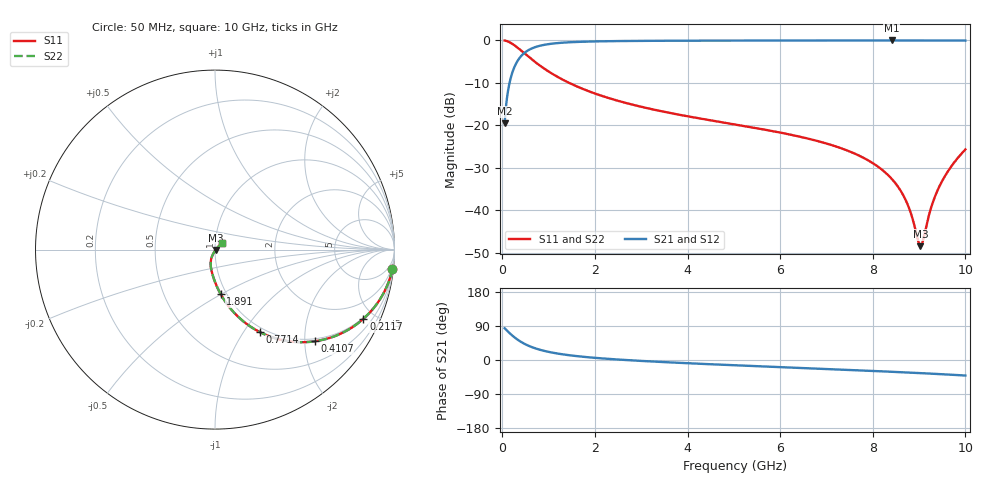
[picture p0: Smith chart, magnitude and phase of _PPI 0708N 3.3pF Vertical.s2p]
! S-Parameter data specifications (vertical orientation):
! Substrate: 40-mil Rogers 3003C, Substrate thickness, H=1.016mm, Dielectric constant, Er=3, Conductor thickness, T_mtl=0.043mm, Loss Tangent, Tand=0.003
! PCB Mounting Pad Footprint: Pad width, PadW=2.54mm , Pad length, PadL=0.51mm , Pad gap, PadG (edge-to-edge)=0.71mm , Reference planes=1.73mm apart
! Created Tue Jan 16 08:45:03 2018
# GHz S MA R 50
! 2 Port Network Data from SP1.SP block
! freq  magS11  angS11  magS21  angS21  magS12  angS12  magS22  angS22
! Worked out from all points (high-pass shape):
!   801 points, 50 MHz to 10 GHz, reference 50 ohm
!   highest |S21| = -0.03 dB at 8.408 GHz (marker M1); lowest = -19.5 dB at 50 MHz (marker M2)
!   |S21| within 3 dB of the highest: 470.5 MHz to end of sweep
!   lowest |S11| = -48.5 dB at 9.03 GHz (marker M3), VSWR 1.01, Z = 50.3 - j0.231 ohm
!   |S11| at or under -10 dB: 1.439 GHz to end of sweep
!   |S22| runs from -48.5 to 0.0 dB; largest |S21 - S12| = 0
!   S11 on the Smith chart (normalised r, x): 50 MHz: 1, -18; 211.7 MHz: 0.94, -4.32; 410.7 MHz: 0.94, -2.23; 771.4 MHz: 0.94, -1.19; 1.891 GHz: 0.94, -0.49; 10 GHz: 1.08, +0.08
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0.05  0.9944 -6.3  0.1054 83.7  0.1054 83.7  0.9944 -6.3
0.1370625  0.9602 -16.7  0.279 73.2  0.279 73.2  0.9602 -16.7
0.2116875  0.9123 -25.0  0.4092 65.0  0.4092 65.0  0.9123 -25.0
0.4106875  0.7545 -42.6  0.6559 47.3  0.6559 47.3  0.7545 -42.6
0.771375  0.5234 -61.5  0.8514 28.5  0.8514 28.5  0.5234 -61.5
1.156937  0.381 -72.1  0.9237 17.8  0.9237 17.8  0.381 -72.1
1.716625  0.2708 -80.9  0.9616 8.9  0.9616 8.9  0.2708 -80.9
1.89075  0.2485 -82.9  0.9675 6.9  0.9675 6.9  0.2485 -82.9
3.370812  0.1487 -94.3  0.9873 -4.8  0.9873 -4.8  0.1487 -94.3
5.025  0.1021 -102.9  0.9927 -13.9  0.9927 -13.9  0.1021 -102.9
6.691625  0.06767 -110.2  0.9951 -22.2  0.9951 -22.2  0.06767 -110.2
7.699063  0.04403 -113.7  0.9959 -27.3  0.9959 -27.3  0.04403 -113.7
8.345812  0.02539 -113.5  0.9962 -30.7  0.9962 -30.7  0.02539 -113.5
8.408  0.0234 -113.1  0.9962 -31.1  0.9962 -31.1  0.0234 -113.1
8.731375  0.01242 -106.6  0.9961 -32.9  0.9961 -32.9  0.01242 -106.6
8.980125  0.004338 -65.5  0.9959 -34.3  0.9959 -34.3  0.004338 -65.5
9.029875  0.003766 -37.5  0.9959 -34.6  0.9959 -34.6  0.003766 -37.5
9.092063  0.004541 -2.4  0.9958 -35.0  0.9958 -35.0  0.004541 -2.4
9.278625  0.01153 33.4  0.9955 -36.1  0.9955 -36.1  0.01153 33.4
9.440312  0.01914 40.0  0.9952 -37.2  0.9952 -37.2  0.01914 40.0
9.7015  0.03311 43.0  0.9944 -38.9  0.9944 -38.9  0.03311 43.0
10  0.05189 43.2  0.993 -41.0  0.993 -41.0  0.05189 43.2
